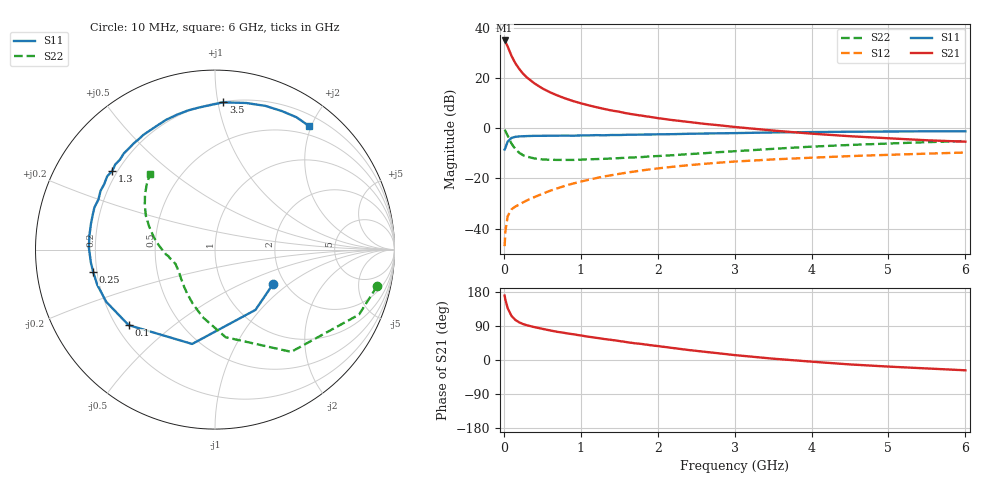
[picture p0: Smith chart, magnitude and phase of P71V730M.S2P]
! SIEMENS Small Signal Semiconductors
! BFP196
! Si NPN RF Bipolar Junction Transistor in SOT143
! VCE = 1.75 V  IC = 30 mA
! Common Emitter S-Parameters:  May  1996
# GHz  S  MA  R  50
!  f  S11  S21  S12  S22
! GHz  MAG  ANG  MAG  ANG  MAG  ANG  MAG  ANG
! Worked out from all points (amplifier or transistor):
!   36 points, 10 MHz to 6 GHz, reference 50 ohm
!   highest |S21| = 34.9 dB at 10 MHz (marker M1)
!   |S21| within 3 dB of that: start of sweep to 57.55 MHz
!   unconditionally stable (mu >= 1): 530.6 MHz to 4.192 GHz
!   at 250 MHz: K = 0.74, MSG = 25.6 dB, |S12| = -29.5 dB
!   at 1.4 GHz: K = 1.10, MAG = 11.0 dB, |S12| = -18.7 dB
!   at 6 GHz: K = 0.99, MSG = 2.2 dB, |S12| = -9.7 dB
!   S11 on the Smith chart (normalised r, x): 10 MHz: 1.74, -0.77; 100 MHz: 0.25, -0.36; 250 MHz: 0.18, -0.09; 1.3 GHz: 0.18, +0.33; 3.5 GHz: 0.21, +1.04; 6 GHz: 0.36, +1.96
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0.01  0.376 -30.6  55.41 170.0  0.0045 81.8  0.9259 -12.7
0.02  0.4046 -56.1  52.29 159.3  0.0088 73.8  0.8803 -24.3
0.05  0.5409 -103.6  41.83 136.6  0.0178 55.6  0.7105 -53.3
0.1  0.6391 -138.8  27.32 116.1  0.0243 45.2  0.4917 -83.1
0.15  0.6721 -154.3  19.49 105.7  0.0277 43.0  0.3818 -100.5
0.2  0.6847 -163.3  15.05 99.3  0.0301 44.6  0.3239 -112.8
0.25  0.69 -169.6  12.11 94.8  0.0334 46.2  0.2898 -122.3
0.3  0.6953 -174.1  10.19 91.7  0.0366 49.0  0.2716 -128.8
0.4  0.7032 178.9  7.728 86.6  0.0427 52.5  0.2494 -139.1
0.5  0.704 173.6  6.18 82.3  0.0495 54.8  0.239 -145.9
0.6  0.706 168.3  5.165 78.1  0.0568 56.5  0.2349 -150.7
0.7  0.7082 164.2  4.443 74.2  0.0639 57.3  0.2336 -154.2
0.9  0.7069 156.8  3.459 67.9  0.0792 57.5  0.2335 -159.6
1.1  0.717 149.4  2.848 61.5  0.0939 56.8  0.2397 -163.1
1.3  0.721 142.5  2.417 55.5  0.1095 54.8  0.2453 -166.4
1.7  0.7408 130.0  1.856 44.2  0.1374 50.7  0.2623 -172.0
2.2  0.7594 116.5  1.442 31.6  0.1709 44.3  0.2899 -178.7
2.8  0.7897 101.0  1.14 17.5  0.2061 36.1  0.3335 171.5
3.5  0.8218 86.8  0.896 3.5  0.2389 26.6  0.3877 160.9
4.5  0.8485 70.7  0.691 -11.7  0.2781 14.9  0.4631 147.6
5.5  0.8659 58.4  0.574 -22.3  0.3113 4.1  0.5263 136.3
6  0.8653 52.8  0.538 -27.2  0.3277 -1.6  0.5548 130.7
